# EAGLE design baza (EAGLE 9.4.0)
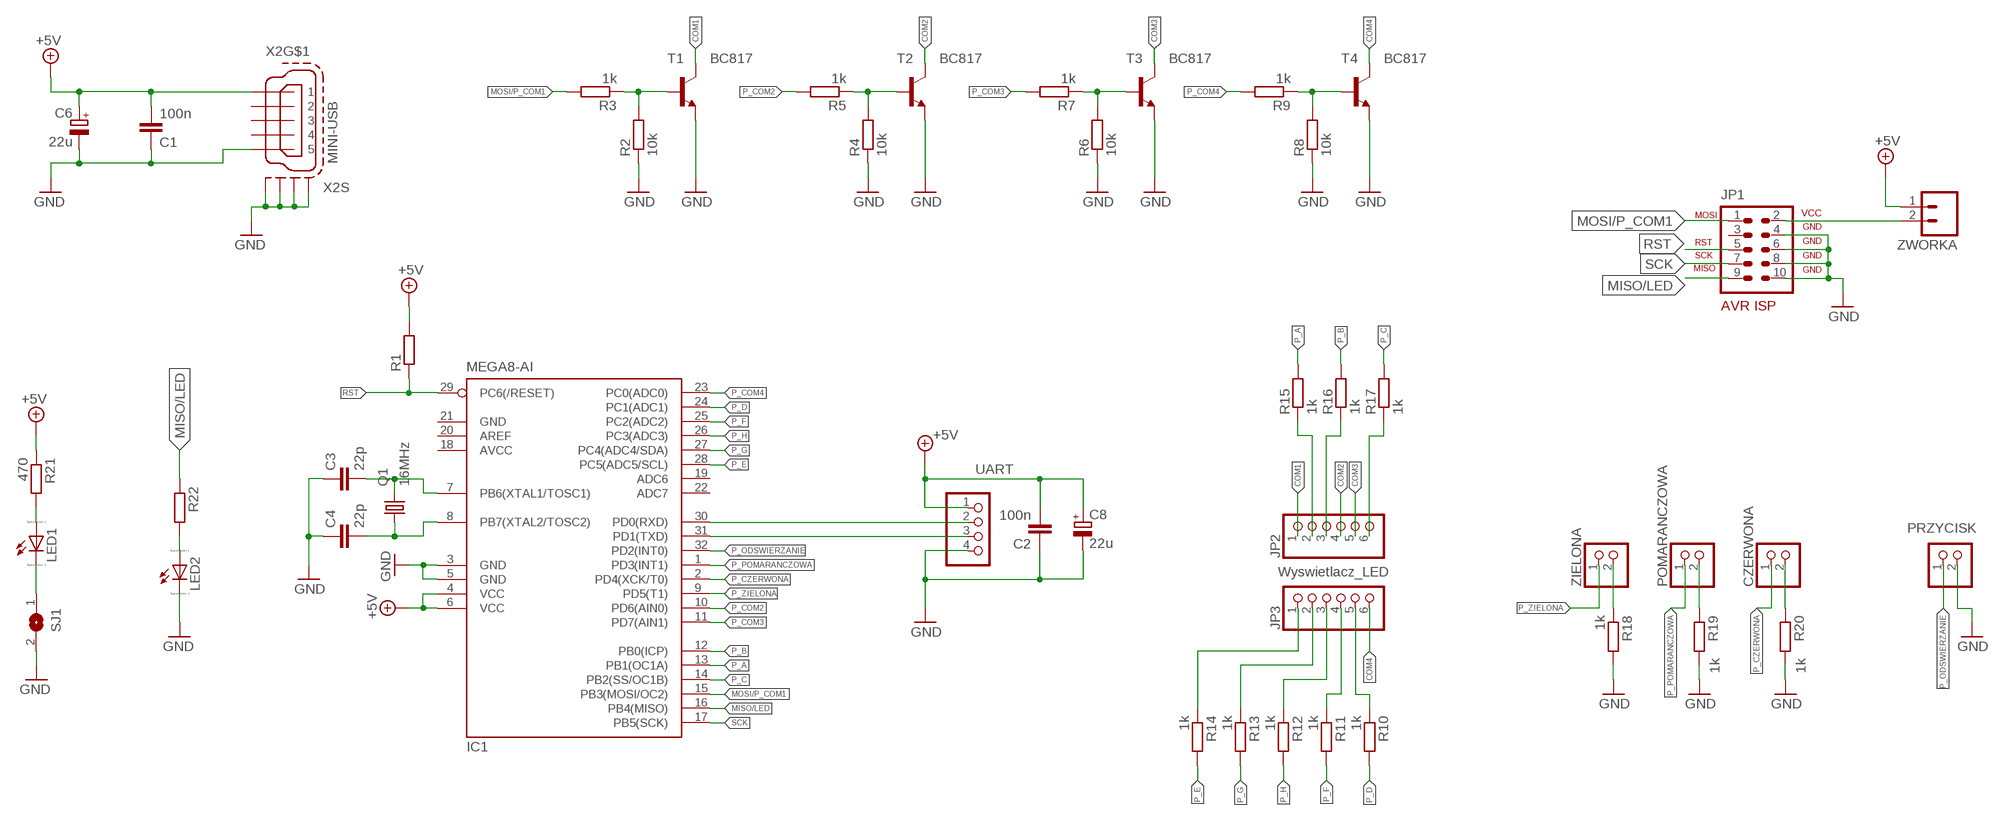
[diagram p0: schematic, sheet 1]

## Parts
C1  100n  C-EUC1206  [C1206]
C2  100n  C-EUC1206  [C1206]
C3  22p  C-EUC1206  [C1206]
C4  22p  C-EUC1206  [C1206]
C6  22u  CPOL-EUSMCB  [SMC_B]
C8  22u  CPOL-EUSMCB  [SMC_B]
CZERWONA  PINHD-1X2  [1X02]
IC1  MEGA8-AI  [TQFP32-08]
JP1  AVR-ISP-10  [AVR-ISP-10]
JP2  PINHD-1X6  [1X06]
JP3  PINHD-1X6  [1X06]
LED1  LED_E  [LED_1206]
LED2  LED_E  [LED_1206]
POMARANCZOWA  PINHD-1X2  [1X02]
PRZYCISK  PINHD-1X2  [1X02]
Q1  16MHz  KX-KS  [11.4X4.5]
R1  R-EU_M1206  [M1206]
R2  10k  R-EU_M1206  [M1206]
R3  1k  R-EU_M1206  [M1206]
R4  10k  R-EU_M1206  [M1206]
R5  1k  R-EU_M1206  [M1206]
R6  10k  R-EU_M1206  [M1206]
R7  1k  R-EU_M1206  [M1206]
R8  10k  R-EU_M1206  [M1206]
R9  1k  R-EU_M1206  [M1206]
R10  1k  R-EU_M1206  [M1206]
R11  1k  R-EU_M1206  [M1206]
R12  1k  R-EU_M1206  [M1206]
R13  1k  R-EU_M1206  [M1206]
R14  1k  R-EU_M1206  [M1206]
R15  1k  R-EU_M1206  [M1206]
R16  1k  R-EU_M1206  [M1206]
R17  1k  R-EU_M1206  [M1206]
R18  1k  R-EU_M1206  [M1206]
R19  1k  R-EU_M1206  [M1206]
R20  1k  R-EU_M1206  [M1206]
R21  470  R-EU_R1206  [R1206]
R22  470  R-EU_R1206  [R1206]
SJ1  SJ  [SJ]
T1  BC817  BC847  [SOT23]
T2  BC817  BC847  [SOT23]
T3  BC817  BC847  [SOT23]
T4  BC817  BC847  [SOT23]
UART  PINHD-1X4  [1X04]
X2  MINI-USB  MINI-USB-SCHIELD-32005-301  [32005-301]
ZIELONA  PINHD-1X2  [1X02]
ZWORKA  M02  [02P]

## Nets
+5V: C1.2 C2.2 C6.+ C8.+ IC1.4(VCC) IC1.6(VCC) R1.2 R21.1 UART.1 X2.1 ZWORKA.1
COM1: JP2.1 T1.3(C)
COM2: JP2.4 T2.3(C)
COM3: JP2.5 T3.3(C)
COM4: JP3.6 T4.3(C)
GND: C1.1 C2.1 C3.1 C4.1 C6.- C8.- IC1.3(GND) IC1.5(GND) JP1.4 JP1.6 JP1.8 JP1.10 LED2.C PRZYCISK.2 R2.1 R4.1 R6.1 R8.1 R18.2 R19.2 R20.2 SJ1.2 T1.2(E) T2.2(E) T3.2(E) T4.2(E) UART.4 X2.5 X2.M1(S:S1) X2.M2(S:S2) X2.M3(S:S3) X2.M4(S:S4)
MISO/LED: IC1.16(PB4(MISO)) JP1.9 R22.1
MOSI/P_COM1: IC1.15(PB3(MOSI/OC2)) JP1.1 R3.2
N$1: C3.2 IC1.7(PB6(XTAL1/TOSC1)) Q1.2
N$2: C4.2 IC1.8(PB7(XTAL2/TOSC2)) Q1.1
N$3: LED1.A R21.2
N$4: CZERWONA.2 R20.1
N$5: JP2.2 R15.1
N$6: JP2.3 R16.1
N$7: POMARANCZOWA.2 R19.1
N$8: R18.1 ZIELONA.2
N$9: JP2.6 R17.1
N$10: JP3.1 R14.1
N$11: JP3.2 R13.1
N$12: JP3.3 R12.1
N$13: JP3.4 R11.1
N$14: JP3.5 R10.1
N$15: JP1.2 ZWORKA.2
N$16: R2.2 R3.1 T1.1(B)
N$17: R4.2 R5.1 T2.1(B)
N$18: R6.2 R7.1 T3.1(B)
N$19: R8.2 R9.1 T4.1(B)
N$20: LED1.C SJ1.1
N$21: LED2.A R22.2
P_A: IC1.13(PB1(OC1A)) R15.2
P_B: IC1.12(PB0(ICP)) R16.2
P_C: IC1.14(PB2(SS/OC1B)) R17.2
P_COM2: IC1.10(PD6(AIN0)) R5.2
P_COM3: IC1.11(PD7(AIN1)) R7.2
P_COM4: IC1.23(PC0(ADC0)) R9.2
P_CZERWONA: CZERWONA.1 IC1.2(PD4(XCK/T0))
P_D: IC1.24(PC1(ADC1)) R10.2
P_E: IC1.28(PC5(ADC5/SCL)) R14.2
P_F: IC1.25(PC2(ADC2)) R11.2
P_G: IC1.27(PC4(ADC4/SDA)) R13.2
P_H: IC1.26(PC3(ADC3)) R12.2
P_ODSWIERZANIE: IC1.32(PD2(INT0)) PRZYCISK.1
P_POMARANCZOWA: IC1.1(PD3(INT1)) POMARANCZOWA.1
P_ZIELONA: IC1.9(PD5(T1)) ZIELONA.1
RST: IC1.29(PC6(/RESET)) JP1.5 R1.1
RX: IC1.31(PD1(TXD)) UART.3
SCK: IC1.17(PB5(SCK)) JP1.7
TX: IC1.30(PD0(RXD)) UART.2
Unconnected: IC1.19(ADC6) IC1.20(AREF) IC1.22(ADC7) JP1.3 X2.2 X2.3 X2.4

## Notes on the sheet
- Wyswietlacz_LED

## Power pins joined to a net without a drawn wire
AVCC: IC1.18(AVCC)
GND: IC1.21(GND)

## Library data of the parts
C1-C4 = resistor:C-EU: CAPACITOR, European symbol
C6 C8 = resistor:CPOL-EU: POLARIZED CAPACITOR, European symbol
CZERWONA POMARANCZOWA PRZYCISK ZIELONA = pinhead:PINHD-1X2: PIN HEADER
IC1 = atmel:MEGA8: MICROCONTROLLER 8 Kbytes FLASH, 1 kbytes SRAM, 512 bytes EEPROM, USART, 6-channel 10 bit ADC, 2-channel 8 bit ADC Pin compatible with Atmega48, ATMega88, ATMega168 Source: avr.lbr; MPN: ATMEGA8-16AU; OC_FARNELL: 9171371; OC_NEWARK: 73M8863
JP1 = avr-7:AVR-ISP-10: AVR ISP-10 Serial Programming Header
JP2 JP3 = pinhead:PINHD-1X6: PIN HEADER
LED1 LED2 = eagle-ltspice:LED_E: LED; SPICEMODEL: NONE; SPICEPREFIX: D; SPICETYPE: diode
Q1 = crystal-geyer_V1_0:KX
R1-R14 R18-R22 = resistor:R-EU_: RESISTOR, European symbol
R15-R17 = resistor:R-EU_: RESISTOR, European symbol; SPICEPREFIX: R
SJ1 = jumper:SJ: SMD solder JUMPER
T1-T4 = transistor:BC847: NPN TRANSISTOR
UART = pinhead:PINHD-1X4: PIN HEADER; SPICEPREFIX: E
X2 = con-cypressindustries:MINI-USB-SCHIELD-: MINI USB-B Conector Source: www.cypressindustries.com; OC_FARNELL: unknown; OC_NEWARK: unknown
ZWORKA = con-amp-quick:M02: AMP QUICK CONNECTOR; OC_FARNELL: unknown; OC_NEWARK: unknown

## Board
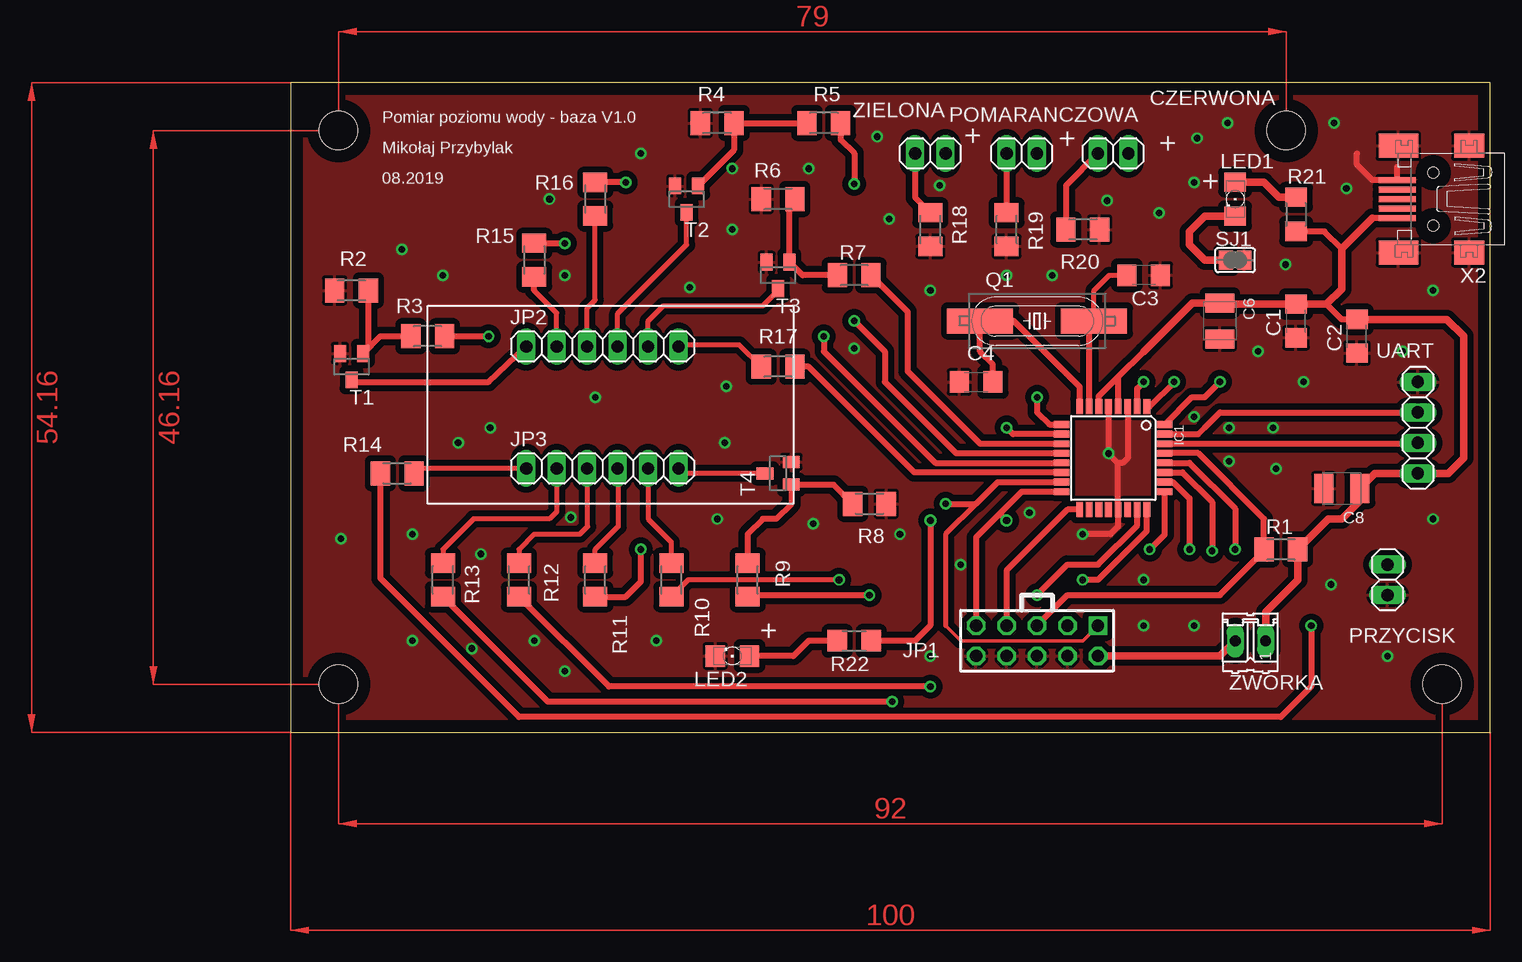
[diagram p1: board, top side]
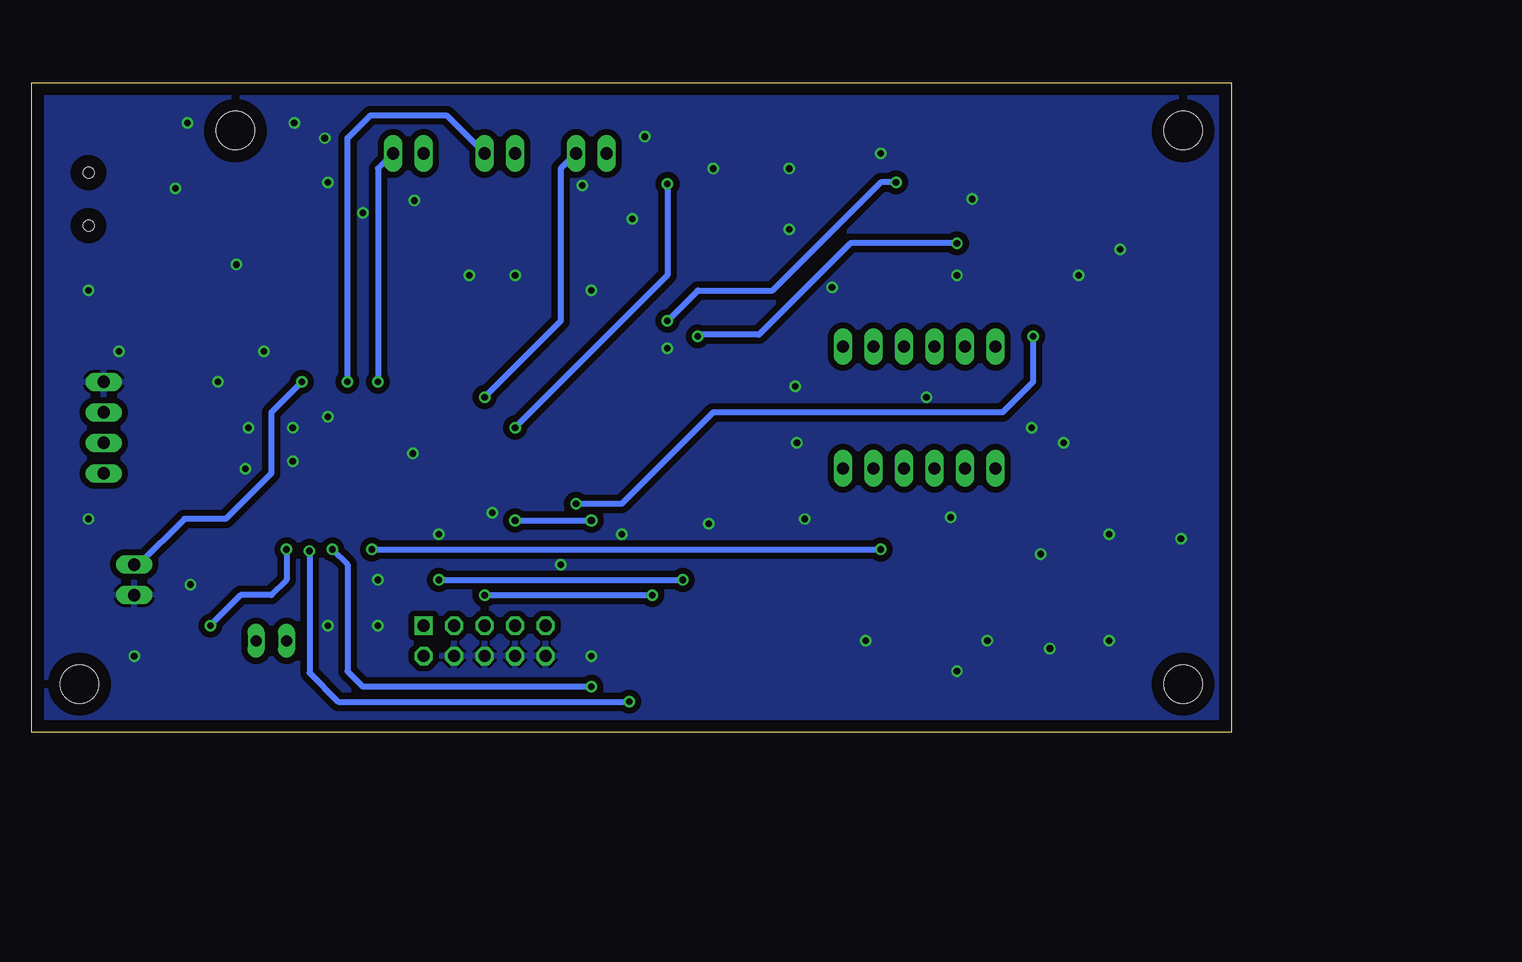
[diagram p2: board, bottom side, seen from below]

Size 100 x 54.16 mm. Coordinates in mm from the lower left corner, seen from the top.
Outline: 0,0 100,0 100,54.16 0,54.16 0,0
Copper layers (1*16): Top 0.035mm / dielectric 1.5mm / Bottom 0.035mm
Design rules "default": minimum track width 6mil, minimum drill 0.35mm, track to track 6mil, track to pad 6mil, pad to pad 6mil, via to via 6mil, smd to smd 6mil, copper to edge 40mil, drill to drill 6mil, minimum pad ring 10mil, minimum via ring 8mil, stop-mask expansion 4mil, vias tented up to drill 0mil, thermal gap 10mil
Holes 3.2 mm at 4,50.16 83,50.16 96,4 4,4

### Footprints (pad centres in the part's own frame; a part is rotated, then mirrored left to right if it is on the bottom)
C1206 = smd 1.6 x 1.8: 1 -1.4,0; 2 1.4,0
SMC_B = smd 1.6 x 2.4: + -1.5,0; - 1.5,0
1X02 = drill 1.016 long: 1 -1.27,0; 2 1.27,0
TQFP32-08 = smd 1.27 x 0.559: 1 -4.293,2.8; 2 -4.293,2; 3 -4.293,1.2; 4 -4.293,0.4; 5 -4.293,-0.4; 6 -4.293,-1.2; 7 -4.293,-2; 8 -4.293,-2.8; 17 4.293,-2.8; 18 4.293,-2; 19 4.293,-1.2; 20 4.293,-0.4; 21 4.293,0.4; 22 4.293,1.2; 23 4.293,2; 24 4.293,2.8 | smd 0.559 x 1.27: 9 -2.8,-4.293; 10 -2,-4.293; 11 -1.2,-4.293; 12 -0.4,-4.293; 13 0.4,-4.293; 14 1.2,-4.293; 15 2,-4.293; 16 2.8,-4.293; 25 2.8,4.293; 26 2,4.293; 27 1.2,4.293; 28 0.4,4.293; 29 -0.4,4.293; 30 -1.2,4.293; 31 -2,4.293; 32 -2.8,4.293
AVR-ISP-10 = drill 1.016 square: 1 -5.08,-1.27 | drill 1.016 octagon: 2 -5.08,1.27; 3 -2.54,-1.27; 4 -2.54,1.27; 5 0,-1.27; 6 0,1.27; 7 2.54,-1.27; 8 2.54,1.27; 9 5.08,-1.27; 10 5.08,1.27
1X06 = drill 1.016 long: 1 -6.35,0; 2 -3.81,0; 3 -1.27,0; 4 1.27,0; 5 3.81,0; 6 6.35,0
LED_1206 = smd 1.6 x 1.803: A -1.422,0; C 1.422,0
11.4X4.5 = smd 5.5 x 2.08: 1 -4.75,0; 2 4.75,0
M1206 = smd 1.6 x 2: 1 -1.4,0; 2 1.4,0
R1206 = smd 1.6 x 1.803: 1 -1.422,0; 2 1.422,0
SJ = smd 1.168 x 1.6: 1 -0.762,0; 2 0.762,0
SOT23 = smd 1 x 1.4: 1 -0.95,-1.1; 2 0.95,-1.1; 3 0,1.1
1X04 = drill 1.016 long: 1 -3.81,0; 2 -1.27,0; 3 1.27,0; 4 3.81,0
32005-301 = smd 3.1 x 0.5: 1 3,1.6; 2 3,0.8; 3 3,0; 4 3,-0.8; 5 3,-1.6 | smd 2.5 x 2: M1 -3,-4.45; M2 -3,4.45 | smd 3.3 x 2: M3 2.9,4.45; M4 2.9,-4.45 | hole 0.9: 0,2.2; 0,-2.2
02P = drill 0.914 long: 1 -1.27,0; 2 1.27,0

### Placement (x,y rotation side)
C1  83.82,34.29 90 top
C2  88.9,33.02 90 top
C3  71.12,38.1 180 top
C4  57.15,29.21 0 top
C6  77.47,34.29 270 top
C8  87.63,20.32 180 top
CZERWONA  68.58,48.26 180 top
IC1  68.58,22.86 270 top
JP1  62.23,7.62 180 top
JP2  26,32.16 0 top
JP3  26,22 0 top
LED1  78.74,44.45 270 top
LED2  36.83,6.35 180 top
POMARANCZOWA  60.96,48.26 180 top
PRZYCISK  91.44,12.7 270 top
Q1  62.23,34.29 0 top
R1  82.55,15.24 0 top
R2  5.08,36.83 0 top
R3  11.43,33.02 0 top
R4  35.56,50.8 0 top
R5  44.45,50.8 0 top
R6  40.64,44.45 0 top
R7  46.99,38.1 0 top
R8  48.26,19.05 180 top
R9  38.1,12.7 270 top
R10  31.75,12.7 270 top
R11  25.4,12.7 270 top
R12  19.05,12.7 270 top
R13  12.7,12.7 270 top
R14  8.89,21.59 180 top
R15  20.32,39.37 90 top
R16  25.4,44.45 90 top
R17  40.64,30.48 0 top
R18  53.34,41.91 270 top
R19  59.69,41.91 270 top
R20  66.04,41.91 0 top
R21  83.82,43.18 90 top
R22  46.99,7.62 180 top
SJ1  78.74,39.37 0 top
T1  5.08,30.48 180 top
T2  33.02,44.45 180 top
T3  40.64,38.1 180 top
T4  40.64,21.59 90 top
UART  93.98,25.4 90 top
X2  95.25,44.45 180 top
ZIELONA  53.34,48.26 180 top
ZWORKA  80.01,7.62 180 top

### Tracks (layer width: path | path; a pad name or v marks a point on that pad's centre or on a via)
+5V
  Top 0.508: 68.98,29.61 IC1.4 | 68.98,29.61 71.12,31.75 | 68.98,29.61 67.38,28.01 IC1.6 | X2.1 90.17,42.85 | C2.2 87.63,34.42 86.36,35.69 | 87.63,40.31 86.18,41.76 R21.1
  Top 0.61: ZWORKA.1 81.28,10.03 83.95,12.7 R1.2 86.49,17.78 87.63,17.78 89.13,19.28 C8.+ 90.4,21.59 UART.1 96.52,21.59 97.79,22.86 97.79,33.02 96.39,34.42 C2.2 | C2.2 88.77,34.29 | 71.12,31.75 75.16,35.79 C6.+ 77.57,35.69 C1.2 86.36,35.69 87.63,36.96 87.63,40.31 90.17,42.85 | 88.51,34.42 C2.2
COM1
  Top 0.508: T1.3 5.25,29.21 16.51,29.21 JP2.1
COM2
  Top 0.406: JP2.4 27.27,34.89 33.02,40.64 T2.3
COM3
  Top 0.406: JP2.5 29.81,34.29 31.08,35.56 39.37,35.56 40.64,36.83
  Top 0.508: 40.64,36.83 T3.3
COM4
  Top 0.406: T4.3 32.76,21.59 JP3.6
GND  (via drill 0.55)
  Top 0.508: 68.98,22.46 IC1.21 68.98,17.14 68.34,16.51 v66.04,16.51 | IC1.5 68.18,23.26 68.98,22.46 | IC1.3 69.78,22.86 69.38,22.46 68.98,22.46 | 88.9,48.26 88.9,47.32 90.17,46.05 X2.5 92.25,47.12
  other vias: 50.8,16.51 95.25,36.83 92.71,31.75 95.25,17.78 30.48,7.62 91.44,6.35 53.34,6.35 10.16,7.62 20.32,7.62 10.16,16.51 22.86,5.08 13.97,24.13 25.4,27.94 12.7,38.1 22.86,38.1 29.21,48.26 36.83,41.91 36.83,46.99 43.18,46.99 48.9,49.66 21.59,44.45 59.69,38.1 63.5,38.1 54.1,45.59 68.2,23.24 82.17,21.97 78.23,22.61 78.23,25.4 75.31,26.29 81.92,25.4 84.45,29.21 78.11,50.8 75.56,49.53 87,50.8 80.64,31.75 36.2,24.13 36.32,28.83 33.27,37.08 35.56,17.78 15.11,6.99 15.88,14.86 16.64,25.4 72.39,43.31 46.99,32 71.12,8.89 23.37,17.91 71.12,12.7 61.59,18.29 55.88,13.97 68.07,44.32 53.34,36.83 75.31,45.85 82.93,38.99 49.91,42.8 9.27,40.26 4.19,16.13 43.56,17.4 86.74,12.32 88.01,45.34 75.31,8.89
  pour Top (isolate 0.508): -6.35,64.77 101.6,64.77 101.6,-10.16 -6.35,-10.16
  pour Bottom (isolate 0.508): -1.27,60.96 -1.27,-2.54 101.6,-2.54 101.6,60.96
MISO/LED  (via drill 0.6)
  Top 0.508: 59.19,18.29 57.15,16.25 JP1.9 | 59.19,18.29 60.96,20.06 IC1.16 | v53.34,17.65 53.34,8.89 52.07,7.62 R22.1 | v59.69,17.65 59.19,18.16 59.19,18.29
  Bottom 0.508: v59.69,17.65 v53.34,17.65
MOSI/P_COM1  (via drill 0.55)
  Top 0.305: JP1.1 66.04,7.62 55.88,7.62 54.61,8.89
  Top 0.406: 54.61,8.89 54.61,16.51 57.15,19.05
  Top 0.508: R3.2 v16.51,33.02 | IC1.15 58.96,20.86 57.15,19.05 v54.61,19.05
  Bottom 0.508: v16.51,33.02 16.51,29.21 19.05,26.67 43.18,26.67 50.8,19.05 v54.61,19.05
N$1
  Top 0.406: Q1.2 66.98,36.83 68.25,38.1 C3.2
  Top 0.508: IC1.7 66.58,33.63 66.91,33.96 | 66.58,34.29 66.91,33.96 | 66.91,33.96 66.89,34.2 Q1.2
N$2
  Top 0.508: IC1.8 65.78,28.79 60.28,34.29 Q1.1 57.48,31.75 58.55,30.68 C4.2
N$3
  Top 0.61: LED1.A 81.13,45.87 82.4,44.6 R21.2
N$4
  Top 0.508: R20.1 64.64,45.59 CZERWONA.2
N$5
  Top 0.406: 20.32,36.83 22.19,34.96 JP2.2
  Top 0.508: 20.32,36.83 R15.1
N$6
  Top 0.406: R16.1 25.4,36.05 24.73,35.38 JP2.3
N$7
  Top 0.508: POMARANCZOWA.2 R19.1
N$8
  Top 0.508: ZIELONA.2 52.07,44.58 R18.1
N$9
  Top 0.406: JP2.6 32.51,32.32 37.4,32.32 R17.1
N$10
  Top 0.406: JP3.1 10.7,22 R14.1
N$11
  Top 0.406: JP3.2 22.19,18.38 21.59,17.78 15.24,17.78 12.7,15.24 R13.1
N$12
  Top 0.406: JP3.3 24.77,21.96 24.77,17.14 24.13,16.51 20.32,16.51 19.05,15.24 R12.1
N$13
  Top 0.406: R11.1 25.4,15.24 27.3,17.14 27.3,21.96 JP3.4
N$14
  Top 0.406: R10.1 31.75,15.84 29.81,17.78 JP3.5
N$15
  Top 0.61: ZWORKA.2 77.47,6.35 JP1.2
N$16
  Top 0.508: R2.2 6.48,32.03 T1.1 7.47,33.02 R3.1
N$17
  Top 0.508: R5.1 R4.2 36.96,48.54 T2.1
N$18
  Top 0.508: R6.2 41.59,44 T3.1 42.69,38.1 R7.1
N$19
  Top 0.508: R9.1 38.1,16.51 39.37,17.78 40.47,17.78 41.74,19.05 T4.1 45.27,20.64 R8.2
N$20
  Top 0.61: SJ1.1 76.2,39.37 74.93,40.64 74.93,41.76 76.2,43.03 LED1.C
N$21
  Top 0.508: R22.2 43.18,7.62 41.91,6.35 LED2.A
P_A  (via drill 0.55)
  Top 0.508: R15.2 v22.86,40.77 | v44.45,33.02 44.45,31.75 53.74,22.46 IC1.13
  Bottom 0.508: v22.86,40.77 31.75,40.77 39.37,33.15 44.32,33.15 v44.45,33.02
P_B  (via drill 0.55)
  Top 0.508: v27.94,45.85 R16.2 | v46.99,34.29 49.53,31.75 49.53,29.21 55.48,23.26 IC1.12
  Bottom 0.508: v27.94,45.85 29.21,45.85 38.23,36.83 44.45,36.83 v46.99,34.29
P_C
  Top 0.508: R17.2 43.18,30.48 52,21.66 IC1.14
P_COM2  (via drill 0.55)
  Top 0.508: R5.2 45.85,49.4 46.99,48.26 v46.99,45.72 | v59.69,25.4 60.23,24.86 IC1.10
  Bottom 0.508: v59.69,25.4 46.99,38.1 v46.99,45.72
P_COM3
  Top 0.508: R7.2 51.44,35.05 51.44,30.1 57.47,24.06 IC1.11
P_COM4  (via drill 0.55)
  Top 0.508: R9.2 38.23,11.43 v48.26,11.43 | v62.23,11.43 64.77,13.97 67.31,13.97 70.58,17.24 IC1.23
  Bottom 0.508: v62.23,11.43 v48.26,11.43
P_CZERWONA  (via drill 0.55)
  Top 0.508: IC1.2 70.58,28.67 v71.12,29.21
  Bottom 0.508: CZERWONA.1 71.12,46.99 v71.12,29.21
P_D  (via drill 0.55)
  Top 0.406: v45.72,12.7 33.15,12.7 31.82,11.37
  Top 0.508: 31.82,11.37 R10.2 | v66.04,12.7 67.31,12.7 71.38,16.77 IC1.24
  Bottom 0.508: v66.04,12.7 v45.72,12.7
P_E  (via drill 0.55)
  Top 0.508: IC1.28 74.93,22.46 78.74,18.65 v78.74,15.24 | v85.09,8.89 85.09,3.81 82.55,1.27 19.05,1.27 7.49,12.83 R14.2
  Bottom 0.508: v78.74,15.24 78.74,12.7 80.01,11.43 82.55,11.43 v85.09,8.89
P_F  (via drill 0.55)
  Top 0.508: R11.2 27.94,11.3 29.21,12.57 v29.21,15.24 | v71.63,15.24 72.87,16.48 IC1.25
  Bottom 0.508: v71.63,15.24 v29.21,15.24
P_G  (via drill 0.55)
  Top 0.508: IC1.27 74.35,21.66 76.83,19.18 v76.83,15.11 | v50.16,2.54 21.46,2.54 R13.2
  Bottom 0.508: v76.83,15.11 76.83,4.95 74.42,2.54 v50.16,2.54
P_H  (via drill 0.55)
  Top 0.508: v74.93,15.24 74.93,19.49 73.56,20.86 IC1.26 | v53.34,3.81 26.54,3.81 R12.2
  Bottom 0.508: v74.93,15.24 73.66,13.97 73.66,5.08 72.39,3.81 v53.34,3.81
P_ODSWIERZANIE  (via drill 0.55)
  Top 0.508: IC1.32 75.15,27.94 76.2,27.94 v77.47,29.21
  Bottom 0.508: PRZYCISK.1 91.06,13.97 87.25,17.78 83.82,17.78 80.01,21.59 80.01,26.67 v77.47,29.21
P_POMARANCZOWA  (via drill 0.55)
  Top 0.508: v73.66,29.21 71.6,27.15 IC1.1
  Bottom 0.508: v73.66,29.21 73.66,49.53 71.75,51.44 65.41,51.44 POMARANCZOWA.1
P_ZIELONA  (via drill 0.55)
  Top 0.508: v62.23,27.94 62.23,26.67 63.24,25.66 IC1.9
  Bottom 0.508: ZIELONA.1 55.88,46.99 55.88,34.29 v62.23,27.94
RST
  Top 0.508: JP1.5 64.77,11.43 77.47,11.43 81.15,15.11 R1.1 81.15,17.78 75.67,23.26 IC1.29
RX
  Top 0.406: 75.66,24.86 76.2,25.4
  Top 0.508: IC1.31 75.66,24.86 | 76.2,25.4 77.47,26.67 UART.3
SCK
  Top 0.508: IC1.17 64.77,18.57 59.69,13.49 JP1.7
TX
  Top 0.508: UART.2 93.91,24.06 IC1.30
(copper drawn outside any net)
  shapes: Top area x5

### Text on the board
tPlace: + | + | + | + | +
tNames: Pomiar poziomu wody - baza V1.0 | Mikołaj Przybylak | 08.2019

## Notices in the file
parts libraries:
crystal-geyer_V1_0: Copyright: Geyer-Electronic
